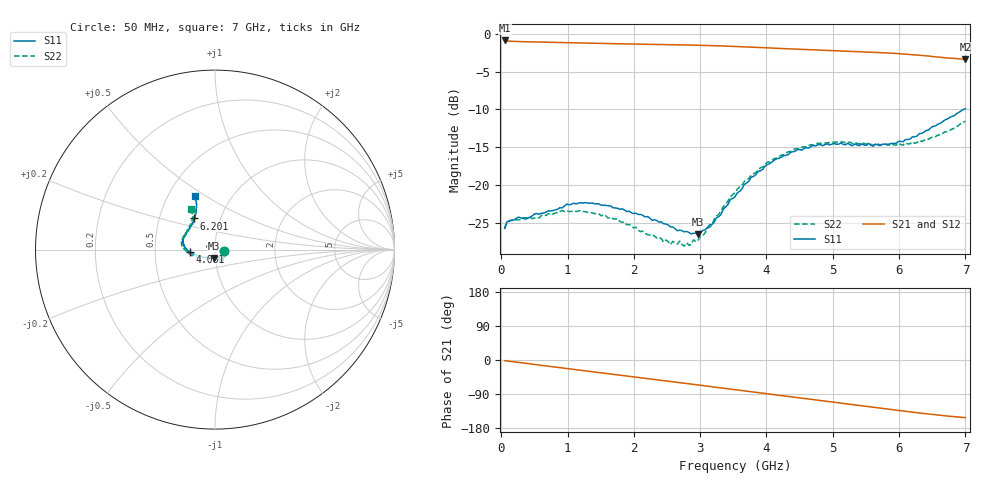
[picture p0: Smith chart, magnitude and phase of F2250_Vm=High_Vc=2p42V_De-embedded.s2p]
! Integrated Device Technology
! Corporate Headquarters
! 6024 Silver Creek Valley Road
! San Jose, CA 95138  USA
! Phone:  1-408-284-8200
! Toll Free:  1-800-223-1366
! Webpage:  http://www.idt.com/
! Timing and RF Division
! 515 Groton Road, Suite 102
! Westford, MA 01886-6024
! Device:  F2250
! Description: Voltage Variable RF Attenuator
! Frequency:  50.0 -  6000.00 MHz
! Package:  3x3 mm Thin QFN Plastic Package: 16 pin
! Ports:  2 RF, 3 DC
!  Pin  1  = GND
!  Pin  2  = NC
!  Pin  3  = RF1  = Port 1
!  Pin  4  = NC
!  Pin  5  = GND
!  Pin  6  = GND
!  Pin  7  = GND
!  Pin  8  = GND
!  Pin  9  = NC
!  Pin 10  = RF2  = Port 2
!  Pin 11  = NC
!  Pin 12  = GND
!  Pin 13  = GND
!  Pin 14  = VCNTRL
!  Pin 15  = VDD
!  Pin 16  = VMODE
! Vcntrl:  2.420 Volts
! Vmode:  +3.300 Volts
! Vdd:  +3.30  Volts
! Current:  1.314 mA
! Data:  The device was measured on a the F2250 evaluation board which has
!  individual transmission lines to the RF pins.  Data was collected
!  using a calibrated network analyzer.  The evaluation board was
!  de-embedded using a TRL calibration technique.
!  The reference plane is the edge of the package pin.
! Misc:  SN 10
!  Action Tracker AT0258
! Date Measured:  2014-11-26
! Date:  2015-10-15  MJV
! Note:
!  Integrated Device Technology supplies this data as a sample of measured
!  data at the package pin for this product.  Your particular data for this
!  product may vary.
!  Data was taken at 25 degrees C.
!  Integrated Device Technology reserves the right to change this data at anytime.
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# GHz S dB R 50
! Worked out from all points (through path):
!   201 points, 50 MHz to 7 GHz, reference 50 ohm
!   highest |S21| = -0.89 dB at 50 MHz (marker M1); lowest = -3.4 dB at 7 GHz (marker M2)
!   group delay of S21, straight-line fit = 61.2 ps
!   lowest |S11| = -26.5 dB at 2.969 GHz (marker M3), VSWR 1.10, Z = 49.1 - j4.62 ohm
!   |S11| at or under -10 dB: start of sweep to 6.967 GHz
!   |S22| runs from -28.1 to -11.6 dB; largest |S21 - S12| = 0.002
!   S11 on the Smith chart (normalised r, x): 50 MHz: 1.11, -0.02; 4.081 GHz: 0.75, -0.02; 6.201 GHz: 0.75, +0.27; 7 GHz: 0.68, +0.45
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0.05  -25.65 -10.7  -0.89 -1.8  -0.89 -1.8  -25.81 -10.9
0.1195  -24.75 -10.2  -0.98 -3.2  -0.98 -3.2  -24.69 -8.9
0.57125  -23.83 -31.3  -1.10 -13.3  -1.10 -13.3  -24.33 -31.4
0.91875  -23.00 -50.1  -1.17 -21.0  -1.17 -21.1  -23.35 -51.0
1.2315  -22.36 -57.9  -1.24 -27.9  -1.24 -27.9  -23.47 -61.5
1.75275  -23.04 -64.9  -1.33 -39.1  -1.33 -39.1  -24.42 -67.8
2.37825  -24.87 -64.5  -1.42 -52.8  -1.42 -52.8  -26.87 -66.8
2.552  -25.51 -69.5  -1.44 -56.7  -1.45 -56.7  -27.86 -73.1
2.691  -25.94 -77.5  -1.47 -59.8  -1.47 -59.8  -27.37 -80.9
2.7605  -26.16 -79.7  -1.48 -61.3  -1.48 -61.3  -28.05 -85.3
2.969  -26.50 -97.8  -1.52 -66.0  -1.52 -66.0  -27.28 -105.0
3.1775  -25.21 -120.9  -1.57 -70.7  -1.57 -70.7  -25.24 -126.8
3.525  -21.54 -152.8  -1.68 -78.5  -1.68 -78.6  -20.97 -148.8
3.76825  -18.97 -164.8  -1.77 -84.0  -1.77 -84.1  -18.70 -159.8
4.081  -16.95 -175.7  -1.90 -91.0  -1.90 -91.0  -16.72 -171.5
4.4285  -15.54 176.0  -2.03 -98.6  -2.04 -98.7  -15.20 178.6
4.7065  -14.76 169.1  -2.13 -104.8  -2.13 -104.8  -14.69 172.9
5.054  -14.60 160.9  -2.26 -112.5  -2.26 -112.5  -14.29 165.9
5.85325  -14.57 135.0  -2.56 -130.0  -2.56 -130.1  -14.69 147.2
6.20075  -13.61 123.5  -2.77 -137.7  -2.77 -137.8  -14.27 138.2
6.54825  -12.18 115.6  -3.04 -144.7  -3.04 -144.9  -13.60 126.9
7  -9.91 110.7  -3.37 -152.1  -3.38 -152.2  -11.56 120.6
